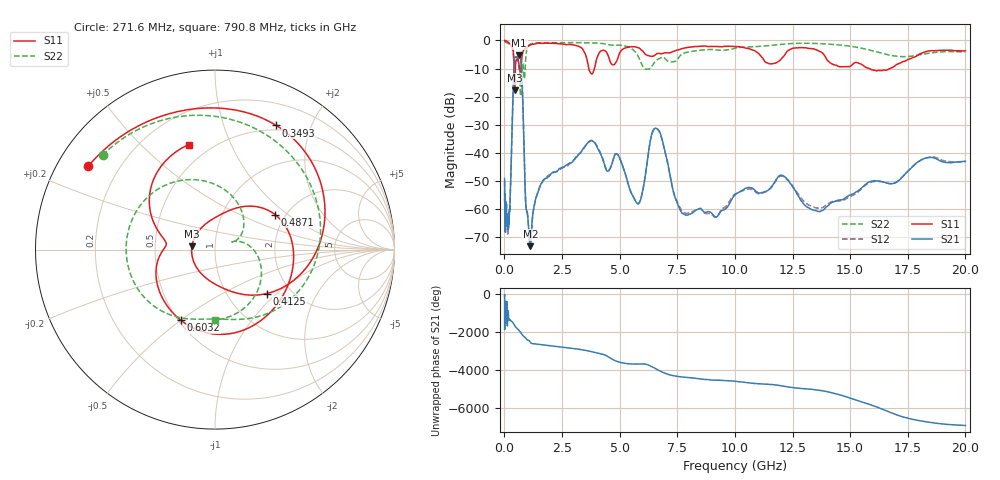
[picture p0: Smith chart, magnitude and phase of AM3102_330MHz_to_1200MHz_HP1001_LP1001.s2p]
! Date/Time: Tue, Sep 11, 2018 5:18 PM
! Network Analyzer: Agilent Technologies E8362B Rev: A.07.50.63
! Sweep from 0.010 to 20.000 GHz, 1601 Points, Sweep Type: LOG
! Power Supply: 4.949 V, 0.001 A
# Hz S DB R 50
!freq MagS11 AngS11 MagS21 AngS21 MagS12 AngS12 MagS22 AngS22
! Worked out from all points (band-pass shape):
!   1601 points, 10 MHz to 20 GHz, reference 50 ohm
!   highest |S21| = -5.31 dB at 632.6 MHz (marker M1); lowest = -73.2 dB at 1.129 GHz (marker M2)
!   |S21| within 3 dB of the highest: 422.6 MHz to 728 MHz (305.4 MHz wide, 53.1 % of centre)
!   lowest |S11| = -17.7 dB at 443 MHz (marker M3), VSWR 1.30, Z = 38.6 + j1.48 ohm
!   |S11| at or under -10 dB: 661.2 MHz to 719.9 MHz (58.75 MHz wide, 8.51 % of centre); 3.663 GHz to 3.905 GHz (242.2 MHz wide, 6.4 % of centre); 15.84 GHz to 16.72 GHz (887.7 MHz wide, 5.45 % of centre)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
!   |S22| runs from -19.7 to -0.2 dB; largest |S21 - S12| = 0.01
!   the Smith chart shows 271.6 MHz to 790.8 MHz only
!   S11 on the Smith chart (normalised r, x): 271.6 MHz: 0.09, +0.30; 349.3 MHz: 0.44, +1.52; 412.5 MHz: 1.52, -0.87; 487.1 MHz: 1.77, +0.81; 603.2 MHz: 0.51, -0.50; 790.8 MHz: 0.38, +0.71
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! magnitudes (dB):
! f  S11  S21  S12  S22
! 10 MHz  0.0  -49.1  -50.2  -0.2
! 35.55 MHz  0.0  -63.6  -63.6  -0.4
! 126.4 MHz  -0.4  -65.6  -64.6  -0.9
! 271.6 MHz  -1.5  -50.7  -51.0  -1.7
! 349.3 MHz  -2.3  -27.1  -27.2  -3.2
! 412.5 MHz  -8.4  -9.9  -10.0  -6.6
! 443 MHz  -17.7  -6.4  -6.5  -8.2
! 447.2 MHz  -17.5  -6.2  -6.3  -8.2
! 487.1 MHz  -8.2  -5.8  -5.8  -6.7
! 603.2 MHz  -7.2  -5.4  -5.6  -7.7
! 632.6 MHz  -8.4  -5.3  -5.4  -9.7
! 705.6 MHz  -11.0  -6.6  -6.6  -19.7
! 790.8 MHz  -4.4  -19.6  -19.6  -8.1
! 920.7 MHz  -2.8  -57.2  -57.5  -6.9
! 1.129 GHz  -1.6  -73.2  -72.8  -1.3
! 1.59 GHz  -1.0  -51.0  -51.1  -0.8
! 3.775 GHz  -11.8  -35.7  -35.6  -0.8
! 5.652 GHz  -2.3  -56.6  -56.6  -3.8
! 6.58 GHz  -4.9  -31.2  -31.4  -7.2
! 7.92 GHz  -2.5  -62.1  -61.5  -4.2
! 13.68 GHz  -3.9  -60.9  -59.6  -1.1
! 20 GHz  -3.6  -42.9  -43.3  -4.1
